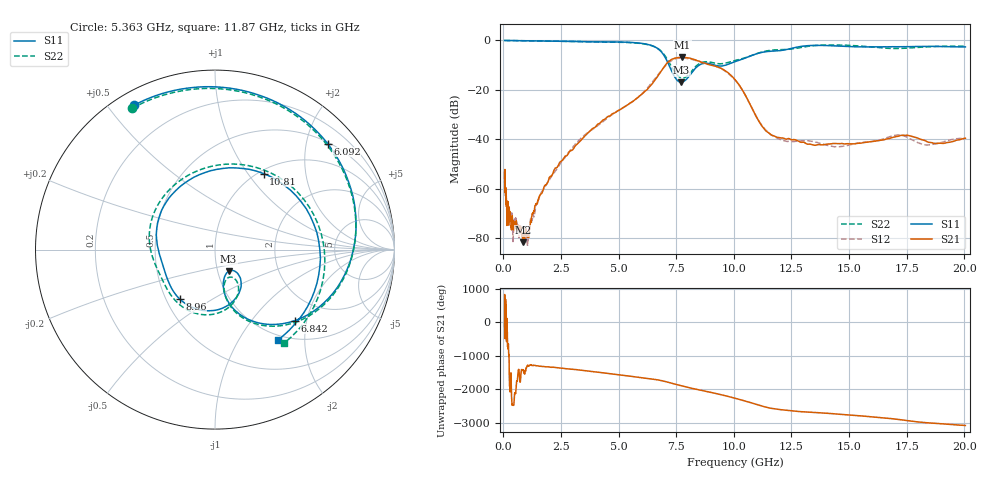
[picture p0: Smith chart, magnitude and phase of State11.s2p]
# Hz S DB R 50
!freq MagS11 AngS11 MagS21 AngS21 MagS12 AngS12 MagS22 AngS22
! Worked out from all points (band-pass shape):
!   1601 points, 50 MHz to 20.05 GHz, reference 50 ohm
!   highest |S21| = -6.82 dB at 7.771 GHz (marker M1); lowest = -81.8 dB at 858.7 MHz (marker M2)
!   |S21| within 3 dB of the highest: 7.04 GHz to 8.936 GHz (1.896 GHz wide, 23.7 % of centre)
!   lowest |S11| = -16.9 dB at 7.713 GHz (marker M3), VSWR 1.33, Z = 56.4 - j13.9 ohm
!   |S11| at or under -10 dB: 7.184 GHz to 8.493 GHz (1.31 GHz wide, 16.7 % of centre); 9.169 GHz to 9.644 GHz (475.3 MHz wide, 5.05 % of centre)
!   |S22| runs from -15.2 to 0.0 dB; largest |S21 - S12| = 0.027
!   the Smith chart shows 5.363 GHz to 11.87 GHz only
!   S11 on the Smith chart (normalised r, x): 5.363 GHz: 0.05, +0.58; 6.092 GHz: 0.53, +2.42; 6.842 GHz: 1.39, -1.71; 8.96 GHz: 0.59, -0.37; 10.81 GHz: 1.05, +1.19; 11.87 GHz: 0.92, -1.50
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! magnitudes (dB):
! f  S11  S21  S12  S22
! 50 MHz  0.0  -55.6  -57.9  0.0
! 135.9 MHz  0.0  -66.2  -66.6  0.0
! 153.3 MHz  0.0  -71.8  -67.2  0.0
! 178 MHz  0.0  -65.9  -67.8  0.0
! 218 MHz  0.0  -74.3  -72.3  0.0
! 250.4 MHz  0.0  -67.6  -70.9  0.0
! 369.6 MHz  0.0  -72.1  -71.8  0.0
! 415.1 MHz  0.0  -75.4  -81.5  0.0
! 533.6 MHz  -0.1  -74.2  -72.7  -0.1
! 858.7 MHz  -0.1  -81.8  -77.8  -0.1
! 1.005 GHz  -0.1  -78.5  -80.7  -0.1
! 2.722 GHz  -0.3  -46.8  -46.7  -0.4
! 5.363 GHz  -0.7  -26.3  -26.3  -0.8
! 6.092 GHz  -1.3  -21.0  -20.8  -1.4
! 6.842 GHz  -4.5  -12.4  -12.3  -4.3
! 7.402 GHz  -14.3  -7.3  -7.6  -12.3
! 7.713 GHz  -16.9  -6.8  -7.1  -15.2
! 7.771 GHz  -16.8  -6.8  -7.1  -15.2
! 8.96 GHz  -9.4  -9.9  -9.6  -8.8
! 10.81 GHz  -6.0  -27.8  -27.8  -6.0
! 11.87 GHz  -4.2  -39.2  -39.5  -3.8
! 20.05 GHz  -2.6  -39.6  -39.5  -2.3
